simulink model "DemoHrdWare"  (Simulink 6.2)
settings: Solver=ode4  SolverMode=SingleTasking  StartTime=0.0  StopTime=Inf  FixedStep=0.001  RelTol=1e-3
libraries: xpclib x2

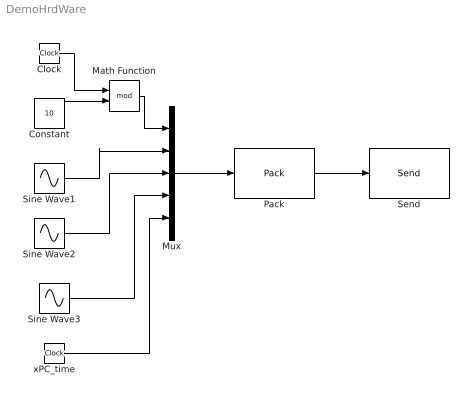
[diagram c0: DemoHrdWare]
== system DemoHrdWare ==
  Clock : Clock
  Constant : Constant  Value=10
  Math Function : Math  Operator=mod
  Mux : Mux  Inputs=5
  Pack : xpclib/UDP/Pack  datatypes={'double'}  byteAlign=1
  Send : xpclib/UDP/Send  ipAddress=132.206.111.72  ipPort=5000  localPort=-1  sampletime=0.02
  Sine Wave1 : Sin  Amplitude=10  Frequency=2*pi*0.25  SampleTime=0
  Sine Wave2 : Sin  Amplitude=10  Frequency=2*pi*0.25  Phase=pi/4  SampleTime=0
  Sine Wave3 : Sin  Amplitude=10  Frequency=2*pi*0.25  Phase=pi/2  SampleTime=0
  xPC_time : Clock
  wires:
  Pack/1 -> Send/1
  Mux/1 -> Pack/1
  Sine Wave1/1 -> Mux/2
  Sine Wave2/1 -> Mux/3
  Sine Wave3/1 -> Mux/4
  Math Function/1 -> Mux/1
  Clock/1 -> Math Function/1
  Constant/1 -> Math Function/2
  xPC_time/1 -> Mux/5
